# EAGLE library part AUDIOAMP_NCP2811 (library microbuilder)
NCP2811 Stereo Headphone Amplifier TSSOP-14 - Mouser: 863-NCP2811ADTBR2G
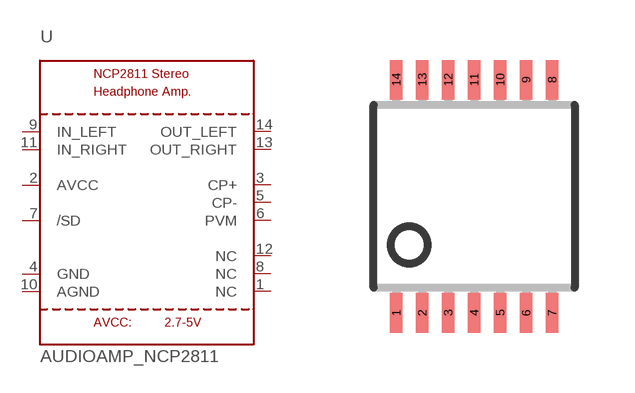
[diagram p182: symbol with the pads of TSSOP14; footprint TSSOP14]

Designator prefix U

## AUDIOAMP_NCP2811  [TSSOP14]
1  NC
2  AVCC
3  CP+
4  GND
5  CP-
6  PVM
7  /SD
8  NC
9  IN_LEFT
10  AGND
11  IN_RIGHT
12  NC
13  OUT_RIGHT
14  OUT_LEFT

## Footprint TSSOP14 (pad centres in mm)
Thin Shrink Small Outline Plastic 14
smd 0.305 x 0.991: 1 -1.95,-2.918; 2 -1.3,-2.918; 3 -0.65,-2.918; 4 0,-2.918; 5 0.65,-2.918; 6 1.3,-2.918; 7 1.95,-2.918; 8 1.95,2.918; 9 1.3,2.918; 10 0.65,2.918; 11 0,2.918; 12 -0.65,2.918; 13 -1.3,2.918; 14 -1.95,2.918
